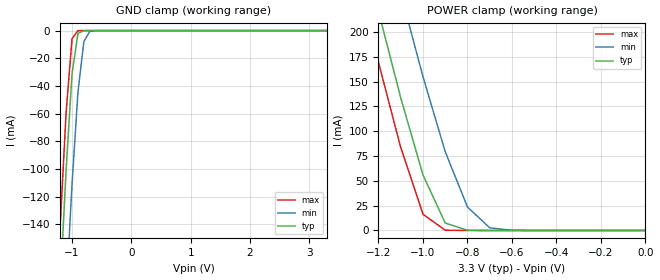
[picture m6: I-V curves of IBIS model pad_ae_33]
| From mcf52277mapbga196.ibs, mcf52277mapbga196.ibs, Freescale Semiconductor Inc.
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|   Model Pad_ae_in
[Model]   pad_ae_33
Model_type   Input
Polarity   Non-Inverting
Vinl =   0.9900V
Vinh =   2.3100V
C_comp   8.5000pF   8.5000pF   8.5000pF
[Temperature Range]   25.0000   0.1500k   -40.0000
[Voltage Range]   3.3000V   3.0000V   3.6000V
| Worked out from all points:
|   GND clamp passes 1 mA (typ) near -0.85 V on its own axis
|   POWER clamp passes 1 mA (typ) near -0.81 V on its own axis
[GND_clamp]
| voltage   I(typ)   I(min)   I(max)
-3.3V     -2.22A     -2.299A    -2.185A
-1.3V     -275.4mA   -367.3mA   -232mA
-1.2V     -185.7mA   -277.6mA   -142mA
-1.1V     -101.3mA   -191.3mA   -59.51mA
-1V       -31.44mA   -111.2mA   -5.922mA
-900mV    -2.018mA   -44.56mA   -54.67uA
-800mV    -44.47uA   -7.861mA   -377.8nA
-700mV    -908.6nA   -617.7uA   -2.61nA
-500mV    -383.6pA   -2.606uA   -5.911pA
3.3V      2.19uA     3.276uA    1.668uA
[POWER_clamp]
| voltage   I(typ)   I(min)   I(max)
-3.3V     2.261A     2.356A     2.218A
-1.3V     311.8mA    418.7mA    260.6mA
-1.2V     220.7mA    327.6mA    169.3mA
-1.1V     133.6mA    239.1mA    83.49mA
-1V       55.96mA    154.9mA    16.31mA
-900mV    7.524mA    79.34mA    253.9uA
-800mV    207.7uA    23.58mA    5.578uA
-700mV    7.758uA    2.697mA    3.649uA
-600mV    3.454uA    189.6uA    3.439uA
0V        2.19uA     2.64uA     2.256uA
